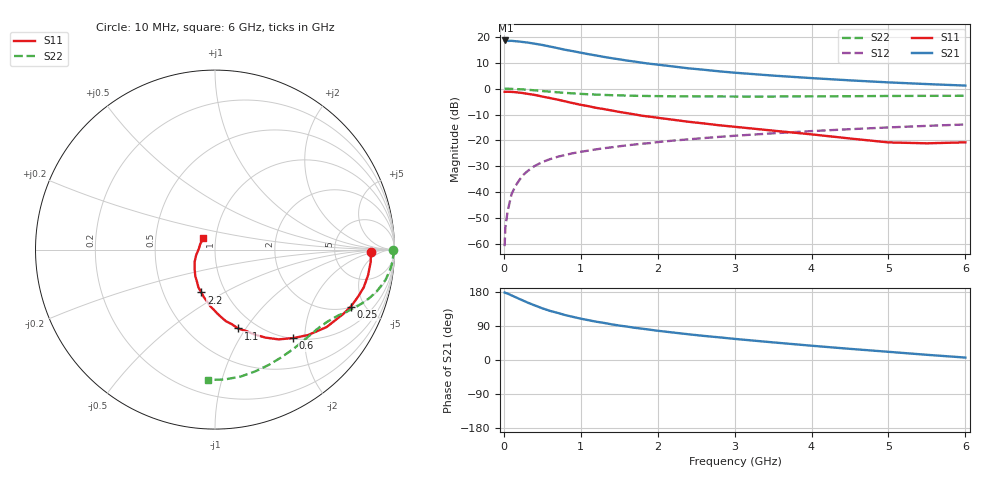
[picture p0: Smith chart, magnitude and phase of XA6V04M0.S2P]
! SIEMENS Discrete & RF Semiconductors
! BFY180
! Si NPN RF Bipolar Junction Transistor in MICRO-X
! VCE = 6 V  IC = 4 mA
! Common Emitter S-Parameters:  May  1997
# GHz  S  MA  R  50
!  f  S11  S21  S12  S22
! GHz  MAG  ANG  MAG  ANG  MAG  ANG  MAG  ANG
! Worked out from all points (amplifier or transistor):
!   36 points, 10 MHz to 6 GHz, reference 50 ohm
!   highest |S21| = 18.6 dB at 20 MHz (marker M1)
!   |S21| within 3 dB of that: start of sweep to 704 MHz
!   unconditionally stable (mu >= 1): 2.187 GHz to end of sweep
!   at 250 MHz: K = 0.19, MSG = 25.7 dB, |S12| = -33.4 dB
!   at 1.4 GHz: K = 0.84, MSG = 17.2 dB, |S12| = -22.7 dB
!   at 6 GHz: K = 1.06, MAG = 6.1 dB, |S12| = -13.9 dB
!   S11 on the Smith chart (normalised r, x): 10 MHz: 14, -1; 250 MHz: 2.03, -3.95; 600 MHz: 1.01, -1.76; 1.1 GHz: 0.83, -0.92; 2.2 GHz: 0.77, -0.39; 6 GHz: 0.87, +0.12
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0.01  0.8678 -0.8  8.497 178.0  0.0009 88.4  0.9919 -0.2
0.02  0.8683 -1.7  8.547 177.2  0.0021 85.5  0.9968 -0.7
0.05  0.8702 -4.4  8.384 175.1  0.0043 86.5  0.9935 -2.0
0.1  0.865 -9.4  8.407 170.6  0.0091 86.0  0.9899 -4.2
0.2  0.8384 -18.4  8.146 161.3  0.0169 79.7  0.9739 -8.1
0.25  0.8201 -22.9  7.966 156.9  0.0213 77.0  0.9654 -10.0
0.3  0.7979 -26.9  7.814 152.3  0.0249 74.4  0.9521 -11.7
0.4  0.7566 -34.8  7.405 144.2  0.0319 70.7  0.9284 -14.8
0.5  0.7042 -42.5  6.992 136.4  0.0381 66.6  0.8996 -17.6
0.6  0.6581 -48.5  6.521 129.6  0.0433 64.2  0.8743 -19.9
0.8  0.5666 -60.0  5.633 118.4  0.0523 59.9  0.8282 -23.7
1  0.487 -68.9  4.959 109.1  0.06 56.4  0.7929 -26.9
1.1  0.4575 -73.7  4.64 105.1  0.0634 55.4  0.7783 -28.1
1.2  0.4254 -77.4  4.378 101.1  0.0671 54.3  0.7672 -29.5
1.5  0.3551 -88.1  3.687 90.9  0.0768 52.0  0.7404 -33.3
1.7  0.3178 -94.6  3.337 85.1  0.0831 50.8  0.7273 -35.9
2.2  0.2505 -107.8  2.686 72.5  0.0989 47.7  0.712 -42.2
2.8  0.1958 -122.3  2.162 59.8  0.1168 44.3  0.7052 -49.6
3.5  0.1542 -137.6  1.788 46.5  0.1369 39.5  0.7047 -58.5
4.5  0.1087 -164.3  1.446 29.4  0.1645 32.4  0.7145 -71.7
5.5  0.0877 158.8  1.226 13.7  0.1907 24.7  0.7256 -85.8
6  0.0916 134.4  1.146 6.4  0.2029 20.5  0.7273 -92.9
